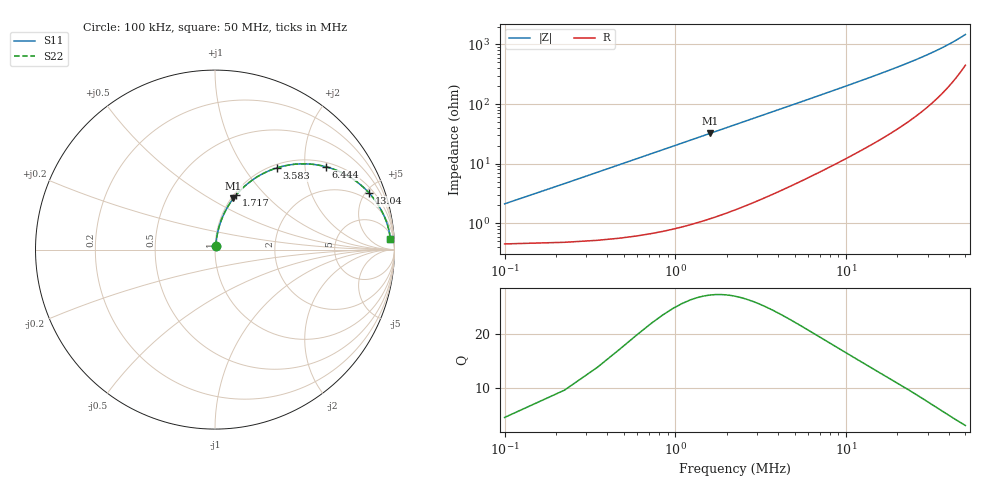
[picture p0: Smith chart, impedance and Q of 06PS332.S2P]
! Coilcraft 0603PS-332 Power Chip Inductor
! 19 February 2003
# MHZ S MA R 50
!Freq  MagS11  AngS11  MagS21  AngS21  MagS12  AngS12  MagS22  AngS22
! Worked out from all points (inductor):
!   403 points, 100 kHz to 50 MHz, reference 50 ohm
!   read as one part in series: L = 3.25 uH near 348.8 kHz
!   highest Q = 27 at 1.593 MHz (marker M1), where L = 3.21 uH
!   S11 on the Smith chart (normalised r, x): 100 kHz: 1.01, +0.04; 1.717 MHz: 1.03, +0.69; 3.583 MHz: 1.06, +1.44; 6.444 MHz: 1.13, +2.58; 13.04 MHz: 1.37, +5.27; 50 MHz: 10, +28
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0.1  0.02111 76.6  0.9953 -1.2  0.9953 -1.2  0.02111 76.6
0.2244  0.04613 81.4  0.9942 -2.6  0.9942 -2.6  0.04613 81.4
0.4732  0.09579 81.2  0.9898 -5.5  0.9898 -5.5  0.09579 81.2
0.5976  0.1203 80.2  0.9867 -6.9  0.9867 -6.9  0.1203 80.2
0.722  0.1444 79.1  0.9829 -8.3  0.9829 -8.3  0.1444 79.1
0.8464  0.1683 77.9  0.9786 -9.7  0.9786 -9.7  0.1683 77.9
1.0952  0.2149 75.4  0.9683 -12.4  0.9683 -12.4  0.2149 75.4
1.5928  0.3028 70.3  0.9419 -17.6  0.9419 -17.6  0.3028 70.3
1.7172  0.3236 69.0  0.9344 -18.9  0.9344 -18.9  0.3236 69.0
2.0904  0.3829 65.4  0.9097 -22.5  0.9097 -22.5  0.3829 65.4
2.588  0.4544 60.8  0.8737 -27.0  0.8737 -27.0  0.4544 60.8
3.5832  0.5724 52.8  0.797 -34.9  0.797 -34.9  0.5724 52.8
4.8272  0.6798 44.7  0.7037 -42.8  0.7037 -42.8  0.6798 44.7
6.4444  0.7718 36.7  0.5986 -50.4  0.5986 -50.4  0.7718 36.7
8.4348  0.8403 29.8  0.4972 -57.0  0.4972 -57.0  0.8403 29.8
10.5496  0.8836 24.6  0.4165 -61.9  0.4165 -61.9  0.8836 24.6
13.0376  0.9143 20.2  0.3464 -65.8  0.3464 -65.8  0.9143 20.2
16.7696  0.9402 15.8  0.273 -69.6  0.273 -69.6  0.9402 15.8
25.1044  0.9646 10.2  0.1779 -73.5  0.1779 -73.5  0.9646 10.2
33.4392  0.9735 7.1  0.1249 -74.2  0.1249 -74.2  0.9735 7.1
41.774  0.9769 5.1  0.09048 -72.7  0.09048 -72.7  0.9769 5.1
50  0.9778 3.6  0.06639 -68.6  0.06639 -68.6  0.9778 3.6
